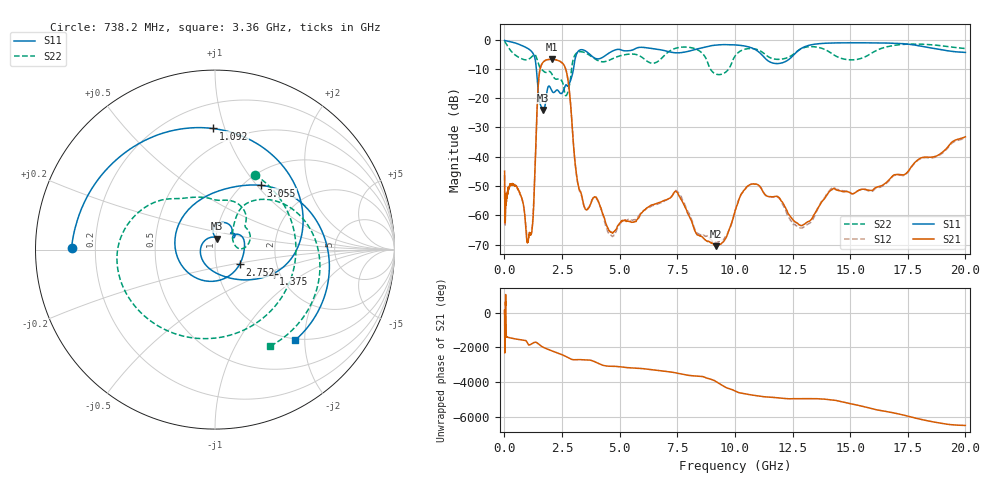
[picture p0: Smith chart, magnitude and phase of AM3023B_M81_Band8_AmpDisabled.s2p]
!Agilent Technologies,E8364B,MY43040894,A.07.50.67
!Agilent E8364B: A.07.50.67
!Date: Tuesday, October 27, 2020 10:40:36
!Correction: S11(Full 2 Port(1,2))
!S21(Full 2 Port(1,2))
!S12(Full 2 Port(1,2))
!S22(Full 2 Port(1,2))
!S2P File: Measurements: S11, S21, S12, S22:Log Frequency Sweep
# Hz S  dB  R 50
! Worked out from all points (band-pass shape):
!   3201 points, 10 MHz to 20 GHz, reference 50 ohm
!   highest |S21| = -6.72 dB at 2.05 GHz (marker M1); lowest = -70.5 dB at 9.176 GHz (marker M2)
!   |S21| within 3 dB of the highest: 1.56 GHz to 2.647 GHz (1.086 GHz wide, 51.6 % of centre)
!   lowest |S11| = -24.0 dB at 1.683 GHz (marker M3), VSWR 1.13, Z = 50.9 + j6.28 ohm
!   |S11| at or under -10 dB: 1.387 GHz to 2.999 GHz (1.611 GHz wide, 73.5 % of centre)
!   |S22| runs from -19.1 to -0.6 dB; largest |S21 - S12| = 0.01
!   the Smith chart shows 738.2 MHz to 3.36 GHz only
!   S11 on the Smith chart (normalised r, x): 738.2 MHz: 0.11, +0.01; 1.092 GHz: 0.37, +0.91; 1.375 GHz: 1.86, -0.56; 2.752 GHz: 1.30, -0.22; 3.055 GHz: 1.19, +1.05; 3.36 GHz: 0.97, -1.80
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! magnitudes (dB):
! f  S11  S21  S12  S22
! 10 MHz  -0.3  -44.9  -46.5  -0.7
! 35.55 MHz  -0.4  -62.5  -63.1  -0.9
! 49.22 MHz  -0.4  -53.8  -53.7  -1.0
! 126.1 MHz  -0.5  -52.9  -53.2  -2.0
! 447.2 MHz  -1.1  -49.7  -49.6  -5.1
! 738.2 MHz  -1.9  -53.8  -53.7  -6.5
! 1.092 GHz  -3.4  -66.0  -65.9  -6.5
! 1.233 GHz  -4.6  -62.0  -61.2  -5.5
! 1.375 GHz  -9.1  -33.4  -33.2  -5.8
! 1.59 GHz  -22.6  -9.0  -9.0  -9.9
! 1.683 GHz  -24.0  -7.7  -7.7  -10.6
! 2.05 GHz  -17.4  -6.7  -6.8  -11.6
! 2.752 GHz  -15.9  -13.4  -13.4  -17.9
! 3.055 GHz  -7.1  -41.1  -41.3  -5.3
! 3.36 GHz  -3.4  -53.5  -53.8  -4.2
! 4.63 GHz  -4.2  -65.8  -66.8  -6.7
! 5.639 GHz  -3.3  -62.2  -61.5  -5.0
! 7.428 GHz  -4.5  -51.8  -51.5  -2.9
! 9.176 GHz  -1.9  -70.5  -69.3  -11.8
! 10.63 GHz  -2.6  -49.6  -49.6  -3.0
! 12.95 GHz  -2.7  -63.3  -64.2  -2.9
! 20 GHz  -4.4  -33.2  -33.5  -3.0
